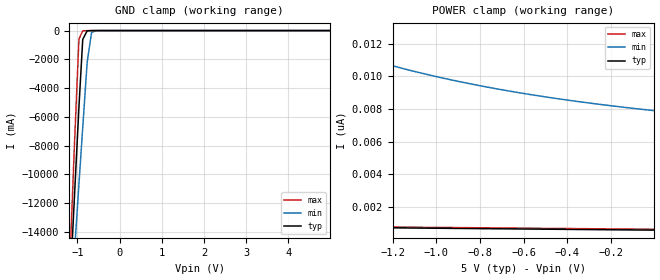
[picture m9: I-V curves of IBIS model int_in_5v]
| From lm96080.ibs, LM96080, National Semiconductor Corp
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[Model] int_in_5v
Model_type Input
Vinh = 2.0V
Vinl = 0.8V
C_comp   1.15pF   1.07pF   1.33pF
[Voltage Range]   5.0V   4.5V   5.5V
[Temperature Range]   25.0   125.0   -40.0
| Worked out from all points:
|   GND clamp passes 1 mA (typ) near -0.63 V on its own axis
[GND Clamp]
-5V       -241.2A    -188.1A    -300.7A
-1.175V   -17.68A    -20.06A    -15.73A
-1.07V    -11.46A    -15.36A    -7.837A
-965mV    -5.314A    -10.69A    -598.6mA
-875mV    -615.6mA   -6.745A    -19.6mA
-770mV    -19.5mA    -2.202A    -2.229mA
-665mV    -1.547mA   -128.1mA   -164.7uA
-560mV    -109.9uA   -8.947mA   -5.848uA
-470mV    -8.714uA   -1.071mA   -206.1nA
4.99V     572.8pA    0A         568.9pA
[POWER Clamp]
-5V       1.262nA    88.04nA    1.197nA
-3.575V   1.022nA    36.25nA    1.035nA
-1.715V   776.5pA    12.97nA    822.5pA
-1.67V    771pA      12.72nA    817.4pA
-1.46V    745.6pA    11.69nA    793.4pA
-1.265V   722.2pA    10.89nA    771.2pA
-1.115V   704.4pA    10.35nA    754.1pA
-905mV    679.5pA    9.706nA    730.2pA
-710mV    656.6pA    9.201nA    707.9pA
-500mV    632pA      8.74nA     684pA
-245mV    602.3pA    8.271nA    654.9pA
-5mV      574.5pA    7.901nA    627.6pA
